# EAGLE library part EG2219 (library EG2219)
SLIDE, 500mA, 15VDC DPDT, On-On Through Hole, Right Angle Source: Datasheet
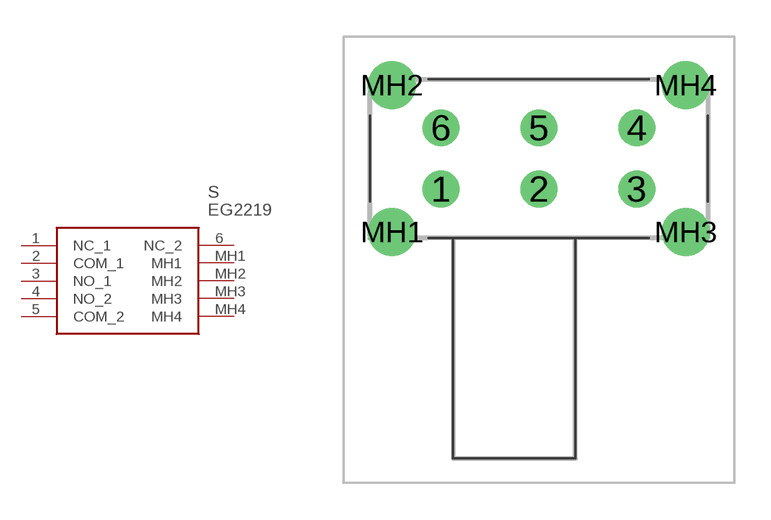
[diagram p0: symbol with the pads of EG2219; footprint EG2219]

Designator prefix S

## EG2219 (Description: SLIDE, 500mA, 15VDC DPDT, On-On Through Hole, Right Angle; Height: 8.5mm; Manufacturer_Name: E-Switch; Manufacturer_Part_Number: EG2219; Mouser_Part_Number: 612-EG2219; Mouser_Price-Stock: https://www.mouser.co.uk/ProductDetail/E-Switch/EG2219?qs=xDsBkp9Lkofjsq7Op0ToJg%3D%3D)  [EG2219]
1  NC_1
2  COM_1
3  NO_1
4  NO_2
5  COM_2
6  NC_2
MH1  MH1
MH2  MH2
MH3  MH3
MH4  MH4

## Footprint EG2219 (pad centres in mm)
EG2219-2
drill 1 pad 1.5: 1 0,0; 2 4,0; 3 8,0; 4 8,2.5; 5 4,2.5; 6 0,2.5
drill 1.3 pad 1.95: MH1 -2,-1.75; MH2 -2,4.25; MH3 10,-1.75; MH4 10,4.25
